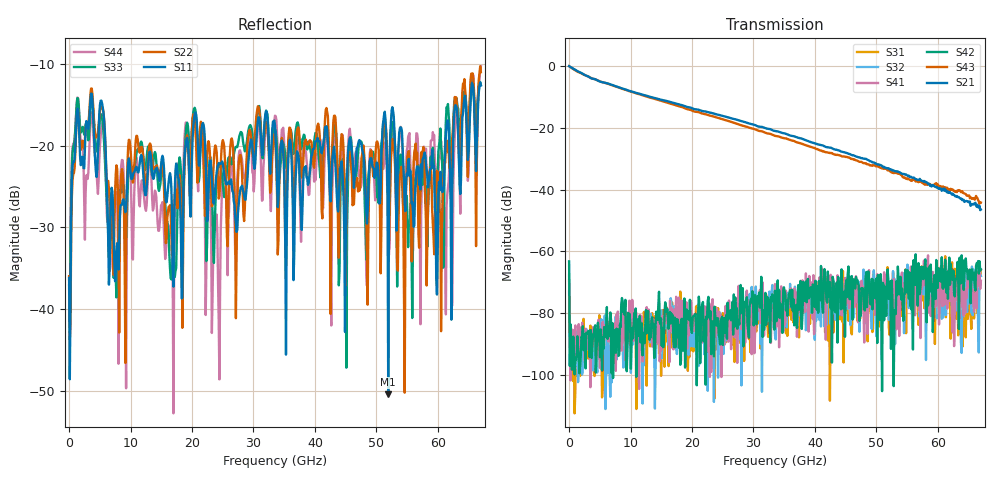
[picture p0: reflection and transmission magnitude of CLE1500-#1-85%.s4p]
!Keysight Technologies,N5247B,US50470101,A.16.20.02
!Date: Thursday, March 13, 2025 10:32:08
!Correction: S11(C  4-Port  )
!S12(C  4-Port  )
!S13(C  4-Port  )
!S14(C  4-Port  )
!S21(C  4-Port  )
!S22(C  4-Port  )
!S23(C  4-Port  )
!S24(C  4-Port  )
!S31(C  4-Port  )
!S32(C  4-Port  )
!S33(C  4-Port  )
!S34(C  4-Port  )
!S41(C  4-Port  )
!S42(C  4-Port  )
!S43(C  4-Port  )
!S44(C  4-Port  )
!S4P File: Measurements: <S11,S12,S13,S14>,
!<S21,S22,S23,S24>,
!<S31,S32,S33,S34>,
!<S41,S42,S43,S44>:
# Hz S  dB  R 50
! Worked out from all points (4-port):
!   601 points, 10 MHz to 67 GHz, reference 50 ohm
!   strongest paths, dB at 10 MHz, 16.76 GHz, 33.51 GHz, 50.25 GHz, 67 GHz:
!     S21: 0.0, -11.8, -21.0, -31.9, -46.5
!     S43: 0.0, -12.3, -22.6, -32.5, -44.2
!     S42: -63.3, -81.4, -72.8, -67.7, -65.9
!     S41: -73.1, -85.9, -70.6, -73.5, -69.6
!     S32: -67.7, -79.3, -87.2, -71.6, -68.0
!     S31: -69.5, -76.6, -78.5, -77.3, -66.2
!   lowest |S11| = -50.4 dB at 51.93 GHz (marker M1), VSWR 1.01, Z = 50 - j0.298 ohm
!   |S11| at or under -10 dB: start of sweep to end of sweep
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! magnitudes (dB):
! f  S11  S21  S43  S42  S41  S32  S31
! 10 MHz  -36.2  0.0  0.0  -63.3  -73.1  -67.7  -69.5
! 3.583 GHz  -13.6  -3.9  -3.9  -86.9  -86.8  -89.1  -91.1
! 7.602 GHz  -35.3  -6.5  -6.6  -92.9  -98.8  -81.1  -87.5
! 20.44 GHz  -16.1  -13.9  -14.7  -80.9  -86.0  -91.0  -89.1
! 24.35 GHz  -22.1  -15.8  -16.8  -87.2  -79.6  -90.5  -86.1
! 51.93 GHz  -50.4  -33.1  -33.8  -68.6  -75.4  -69.4  -73.8
! 67 GHz  -12.6  -46.5  -44.2  -65.9  -69.6  -68.0  -66.2
